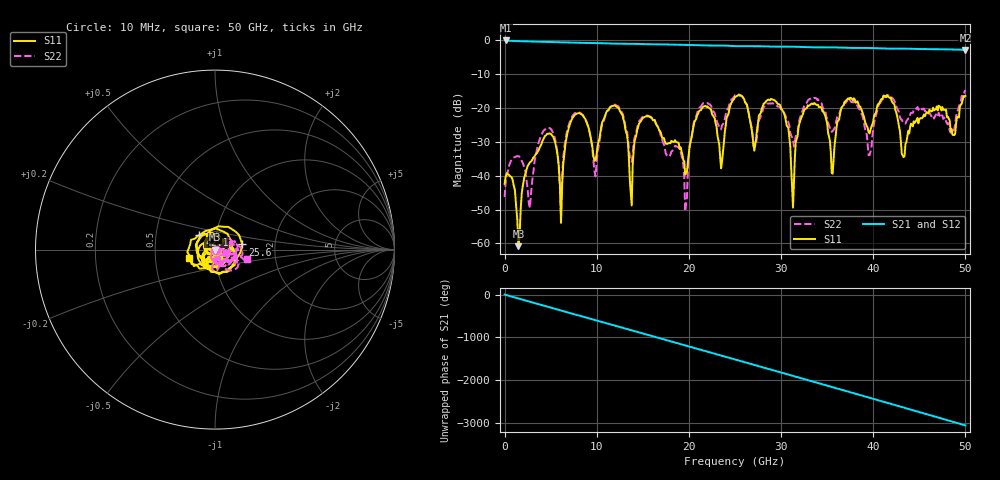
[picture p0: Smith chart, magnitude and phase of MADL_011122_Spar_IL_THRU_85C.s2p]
#	HZ	S	DB	R	50
!Frequency	S11 (dB)	S11-Ang	S21 (dB)	S21-Ang	S12 (dB)	S12-Ang	S22 (dB)	S22-Ang
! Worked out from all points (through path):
!   401 points, 10 MHz to 50 GHz, reference 50 ohm
!   highest |S21| = -0.03 dB at 135 MHz (marker M1); lowest = -2.8 dB at 50 GHz (marker M2)
!   group delay of S21, straight-line fit = 169 ps
!   lowest |S11| = -60.8 dB at 1.51 GHz (marker M3), VSWR 1.00, Z = 49.9 - j0.0728 ohm
!   |S11| at or under -10 dB: start of sweep to end of sweep
!   |S22| runs from -51.2 to -14.7 dB; largest |S21 - S12| = 0.015
!   S11 on the Smith chart (normalised r, x): 10 MHz: 1.01, -0.01; 25.6 GHz: 1.36, +0.08; 42.1 GHz: 0.83, +0.14; 50 GHz: 0.75, -0.08
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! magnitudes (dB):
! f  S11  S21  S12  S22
! 10 MHz  -42.4  0.0  0.0  -46.3
! 135 MHz  -40.1  0.0  0.0  -41.5
! 1.51 GHz  -60.8  -0.2  -0.3  -34.2
! 2.76 GHz  -36.0  -0.3  -0.3  -49.5
! 4.51 GHz  -28.0  -0.5  -0.5  -26.0
! 6.13 GHz  -53.9  -0.6  -0.6  -51.2
! 8.38 GHz  -21.9  -0.7  -0.7  -21.8
! 12.3 GHz  -19.9  -1.0  -1.0  -19.4
! 13.8 GHz  -48.8  -1.0  -1.0  -35.9
! 16.8 GHz  -26.6  -1.2  -1.2  -26.6
! 19.6 GHz  -39.7  -1.3  -1.3  -50.5
! 21.1 GHz  -20.9  -1.4  -1.5  -20.0
! 23.5 GHz  -37.8  -1.5  -1.5  -26.3
! 25.1 GHz  -16.6  -1.7  -1.7  -16.2
! 25.6 GHz  -16.2  -1.7  -1.7  -16.2
! 31.3 GHz  -49.4  -1.9  -1.9  -29.4
! 33.4 GHz  -18.7  -2.1  -2.1  -16.9
! 35.5 GHz  -39.2  -2.1  -2.1  -27.0
! 41.8 GHz  -17.0  -2.5  -2.5  -16.5
! 42.1 GHz  -18.4  -2.5  -2.5  -17.1
! 43.4 GHz  -34.1  -2.4  -2.4  -24.5
! 50 GHz  -16.4  -2.8  -2.9  -14.7
